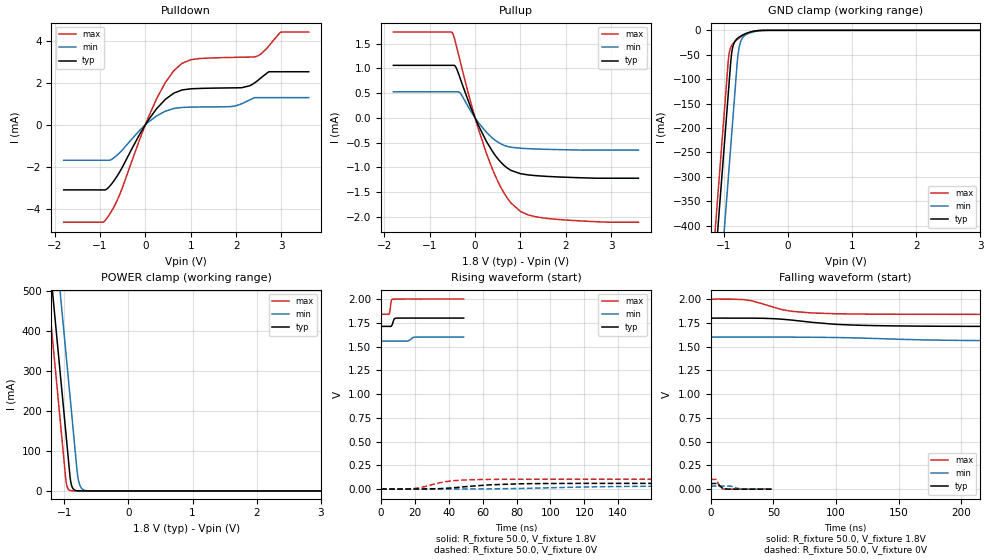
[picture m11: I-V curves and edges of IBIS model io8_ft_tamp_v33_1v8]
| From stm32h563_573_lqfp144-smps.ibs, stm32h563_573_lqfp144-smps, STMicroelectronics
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[Model]   io8_ft_tamp_v33_1v8
Model_type I/O
Polarity   Non-Inverting
Enable   Active-Low
| CAP_THRESHOLD on pad IOFT is "UDTCAPC" :
| Rising=20.0% of vddiom   Falling=80.0% of vddiom
| C_comp min and max val. don't necessarily correlate with the min and max pvt
| but are the smallest and greatest pad capacitance found.
| var   typ   min   max
C_comp   7.54606pF  7.42836pF  7.97687pF
|C_comp_pullup   4.58225pF  4.31295pF  4.49440pF
|C_comp_pulldown   2.96381pF  3.11541pF  3.48247pF
Vinl = 800.0mV
Vinh = 1.0V
Vmeas = 900.0mV   | Reference voltage for timing measurements
Cref  = 50.0pF   | Timing specification test load capacitance value
Rref  = 1.0MOhm   | Timing specification test load resistance value
Vref  = 990.0mV   | Timing specification test load voltage
[Model Spec]
| TIME_THRESHOLD on pin ZIV33SW is "CMOS" :
| Rising=40.0% of VDDV33SW   Falling=60.0% of VDDV33SW
Vinl 699.80000mV 627.80000mV 779.80000mV
Vinh 1.05220V 928.20000mV 1.15620V
| variable   typ   min   max
[Temperature Range] 25.0 125.0 -40.0
| variable   typ   min   max
[Voltage Range] 1.8V 1.6V 2.0V
| variable   typ   min   max
[POWER Clamp Reference] 1.8V 1.6V 2.0V
| variable   typ   min   max
[GND Clamp Reference] 0V 0V 0V
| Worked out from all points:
|   slope of the pulldown table from 0 to 0.27 V, typ, clamps not added: 331 ohm
|   slope of the pullup table from 0 to 0.27 V, typ, clamps not added: 534 ohm
|   GND clamp passes 1 mA (typ) near -0.49 V on its own axis
|   POWER clamp passes 1 mA (typ) near -0.82 V on its own axis
|   rising waveform, R_fixture 50.0, V_fixture 1.8V: 20-80 % time 1.01ns typ, NA min, 690ps max; typ from 1.71 V to 1.8 V
|   falling waveform, R_fixture 50.0, V_fixture 1.8V: 20-80 % time 46.4ns typ, NA min, 28.4ns max; typ from 1.8 V to 1.71 V
|   rising waveform, R_fixture 50.0, V_fixture 0V: 20-80 % time 27.9ns typ, NA min, 15.7ns max; typ from 0 V to 0.059 V
|   falling waveform, R_fixture 50.0, V_fixture 0V: 20-80 % time 3.03ns typ, NA min, 2.21ns max; typ from 0.059 V to 0 V
[POWER Clamp]
-1.8V     1.549A     1.75A      1.43A
-1.26V    630.6mA    832.2mA    511.9mA
-1.24V    596.6mA    798.2mA    477.9mA
-1.18V    494.6mA    696.2mA    375.9mA
-1.06V    290.6mA    492.2mA    171.9mA
-970mV    137.6mA    339.2mA    21.83mA
-920mV    52.59mA    254.2mA    1.812mA
-880mV    11.09mA    186.2mA    247.5uA
-790mV    333.8uA    37.52mA    2.807uA
-750mV    70.36uA    11.69mA    383.6nA
-690mV    6.81uA     2.034mA    19.57nA
3.6V      0A         0A         0A
[GND Clamp]
-1.8V     -1.611A    -1.784A    -1.543A
-1.24V    -659mA     -831.9mA   -591mA
-1.05V    -336mA     -508.9mA   -268mA
-930mV    -132mA     -304.9mA   -64.04mA
-910mV    -98mA      -270.9mA   -44.02mA
-880mV    -50.93mA   -219.9mA   -31.99mA
-840mV    -26.59mA   -151.9mA   -24.84mA
-780mV    -15.91mA   -53.47mA   -17.79mA
-720mV    -10.67mA   -18.29mA   -12.21mA
-600mV    -4.088mA   -5.465mA   -4.221mA
-350mV    -41.3uA    -221.4uA   -10.36uA
3.6V      6.94nA     1.304uA    424.5pA
| variable   typ   min   max
[Pullup Reference] 1.8V 1.6V 2.0V
| variable   typ   min   max
[Pulldown Reference] 0V 0V 0V
[Pullup]
-1.8V     1.061mA    526.5uA    1.732mA
-500mV    1.061mA    526.5uA    1.715mA
-430mV    1.034mA    526.5uA    1.519mA
-330mV    802.5uA    502.8uA    1.148mA
0V        7.53pA     697pA      4.4pA
250mV     -475.1uA   -292.7uA   -718uA
440mV     -751.9uA   -450.5uA   -1.159mA
620mV     -943.6uA   -547uA     -1.488mA
800mV     -1.064mA   -594uA     -1.727mA
1V        -1.128mA   -613.8uA   -1.89mA
1.74V     -1.189mA   -639.1uA   -2.045mA
3.6V      -1.219mA   -651uA     -2.107mA
[Pulldown]
-1.8V     -3.102mA   -1.69mA    -4.639mA
-860mV    -3.077mA   -1.69mA    -4.487mA
-570mV    -2.261mA   -1.338mA   -3.345mA
-120mV    -435uA     -252.8uA   -672.9uA
250mV     768.4uA    423.6uA    1.247mA
630mV     1.508mA    776.9uA    2.582mA
810mV     1.658mA    825.5uA    2.926mA
1.93V     1.756mA    875.9uA    3.208mA
2.43V     2.028mA    1.292mA    3.244mA
2.72V     2.524mA    1.292mA    3.748mA
2.98V     2.524mA    1.292mA    4.412mA
3.6V      2.524mA    1.292mA    4.412mA
[Ramp]
dV/dt_r 35.68178mV/26.50386ns 19.04282mV/50.89389ns 61.70405mV/15.62994ns
dV/dt_f 52.53456mV/45.57689ns 25.57754mV/80.26017ns 96.13671mV/28.11665ns
R_load = 50.0
| Removed startup time: 0s 0s 0s  .
| Removed end time: 48.75ns.
[Rising Waveform]
R_fixture   = 50.0
V_fixture   = 1.8V
V_fixture_min = 1.6V
V_fixture_max = 2.0V
0s        1.712V     1.557V     1.84V
4.65ns    1.712V     1.557V     1.841V
5.15ns    1.712V     1.557V     1.87V
6ns       1.716V     1.557V     1.98V
6.95ns    1.753V     1.557V     1.999V
7.8ns     1.792V     1.557V     1.999V
8.95ns    1.799V     1.557V     2V
15.95ns   1.8V       1.559V     2V
19.9ns    1.8V       1.599V     2V
48.75ns   1.8V       1.6V       2V
| Removed startup time: 0s 0s 0s  .
| Removed end time: 798.75ns.
[Falling Waveform]
R_fixture   = 50.0
V_fixture   = 1.8V
V_fixture_min = 1.6V
V_fixture_max = 2.0V
0s        1.8V       1.6V       2V
26.9ns    1.8V       1.6V       1.995V
32.6ns    1.8V       1.6V       1.982V
54.35ns   1.791V     1.6V       1.898V
62.25ns   1.782V     1.6V       1.877V
80.45ns   1.756V     1.599V     1.855V
100.5ns   1.734V     1.596V     1.846V
146.7ns   1.718V     1.579V     1.841V
244.6ns   1.713V     1.561V     1.84V
798.8ns   1.712V     1.557V     1.84V
| Removed startup time: 0s 0s 0s  .
| Removed end time: 798.7ns.
[Rising Waveform]
R_fixture   = 50.0
V_fixture   = 0V
V_fixture_min = 0V
V_fixture_max = 0V
0s        104.8nV    1.663uV    100.9nV
18.8ns    -41.32uV   -464.3uV   4.477mV
23.1ns    309.1uV    -54.98uV   15.12mV
33.6ns    3.554mV    -22.38uV   61.92mV
40.7ns    10.6mV     17.65uV    83.44mV
48.9ns    23.23mV    254uV      95.15mV
65.2ns    45.01mV    1.523mV    101.6mV
97.8ns    57.86mV    12.47mV    102.7mV
179.3ns   59.41mV    30.48mV    102.8mV
798.7ns   59.47mV    31.74mV    102.8mV
| Removed startup time: 0s 0s 0s  .
| Removed end time: 48.75ns.
[Falling Waveform]
R_fixture   = 50.0
V_fixture   = 0V
V_fixture_min = 0V
V_fixture_max = 0V
0s        59.48mV    31.77mV    102.8mV
4.4ns     59.47mV    31.77mV    102.8mV
5.45ns    58.78mV    31.77mV    72.59mV
7ns       37.65mV    31.77mV    26.06mV
8.85ns    15.17mV    31.77mV    7.014mV
9.95ns    8.427mV    31.77mV    1.962mV
15.95ns   253.2uV    31.92mV    117.4uV
21.7ns    65.49uV    7.981mV    57.73uV
26.9ns    30.29uV    1.503mV    49.75uV
48.75ns   25.14uV    25.02uV    26.22uV
